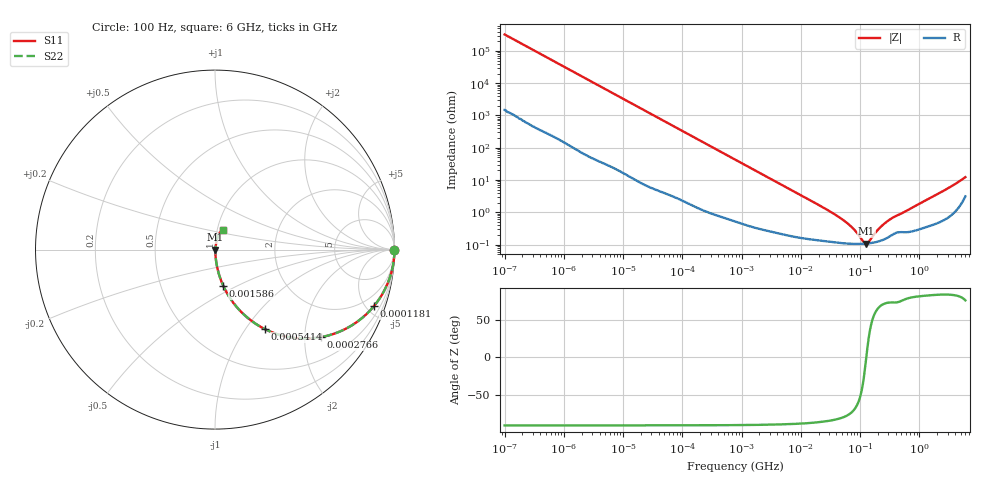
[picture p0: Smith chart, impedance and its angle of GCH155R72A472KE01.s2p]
!Murata Part Number: GCH155R72A472KE01
!These Parameters are Measured in Series Mode Connection
!Data Generated on Mar 13, 2026
!  o--ll--o
!Port1  Port2
!  o------o
!Operation Temp=25[degC], DC Bias Voltage=0[V]
!Freq. Start=100[Hz] Stop=6[GHz] 401[Steps]
# Hz S RI R 50
!Freq.(Hz) S11(Real) S11(Imag) S21(Real) S21(Imag) S12(Real) S12(Imag) S22(Real) S22(Imag)
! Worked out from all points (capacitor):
!   401 points, 100 Hz to 6 GHz, reference 50 ohm
!   read as one part in series: C = 4.9 nF near 109 Hz
!   lowest |Z| = 107 mohm at 127.6 MHz (marker M1)
!   series resonance near 127.4 MHz, so ESL is about 320 pH
!   S11 on the Smith chart (normalised r, x): 100 Hz: open; 118.1 kHz: 1.04, -5.62; 276.6 kHz: 1.02, -2.41; 541.4 kHz: 1.01, -1.23; 1.586 MHz: 1.01, -0.42; 6 GHz: 1.06, +0.24
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100  1 -0.000308  1.5e-06 0.000308  1.5e-06 0.000308  1 -0.000308
2008  0.9999 -0.00613  6.37e-05 0.00613  6.37e-05 0.00613  0.9999 -0.00613
12592  0.9984 -0.0382  0.00165 0.0382  0.00165 0.0382  0.9984 -0.0382
40335  0.9846 -0.1202  0.0154 0.1202  0.0154 0.1202  0.9846 -0.1202
118133  0.8857 -0.3147  0.1143 0.3147  0.1143 0.3147  0.8857 -0.3147
176758  0.7777 -0.4121  0.2223 0.4121  0.2223 0.4121  0.7777 -0.4121
276587  0.5907 -0.4876  0.4093 0.4876  0.4093 0.4876  0.5907 -0.4876
541393  0.2775 -0.4426  0.7225 0.4426  0.7225 0.4426  0.2775 -0.4426
774597  0.1602 -0.3608  0.8398 0.3608  0.8398 0.3608  0.1602 -0.3608
1585629  0.0459 -0.2014  0.9541 0.2014  0.9541 0.2014  0.0459 -0.2014
4246196  0.00847 -0.0788  0.9915 0.0788  0.9915 0.0788  0.00847 -0.0788
1.555665e7  0.00189 -0.0217  0.9981 0.0217  0.9981 0.0217  0.00189 -0.0217
3.482834e7  0.00127 -0.00925  0.9987 0.00925  0.9987 0.00925  0.00127 -0.00925
5.699437e7  0.0011 -0.00493  0.9989 0.00493  0.9989 0.00493  0.0011 -0.00493
8.154455e7  0.00105 -0.00256  0.9989 0.00256  0.9989 0.00256  0.00105 -0.00256
1.166697e8  0.00106 -0.00049  0.9989 0.00049  0.9989 0.00049  0.00106 -0.00049
1.275994e8  0.00107 8.3e-06  0.9989 -8.3e-06  0.9989 -8.3e-06  0.00107 8.3e-06
1.395531e8  0.00109 0.000507  0.9989 -0.000507  0.9989 -0.000507  0.00109 0.000507
2.183701e8  0.0013 0.00313  0.9987 -0.00313  0.9987 -0.00313  0.0013 0.00313
3.124326e8  0.00178 0.00555  0.9982 -0.00555  0.9982 -0.00555  0.00178 0.00555
1.95892e9  0.00567 0.0346  0.9943 -0.0346  0.9943 -0.0346  0.00567 0.0346
6e9  0.043 0.1105  0.957 -0.1105  0.957 -0.1105  0.043 0.1105
